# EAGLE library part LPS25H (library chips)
ST-Micro Piezoresistive pressure sensor
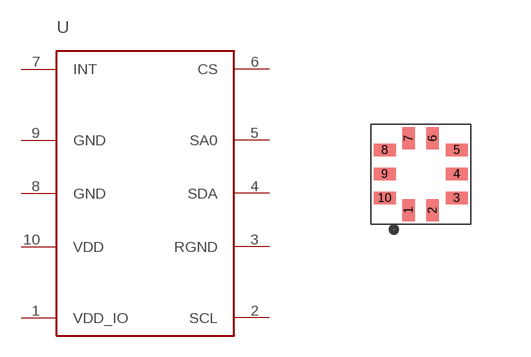
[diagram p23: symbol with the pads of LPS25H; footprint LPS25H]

Designator prefix -

## LPS25H (DIGIKEY: 497-15070-1-ND)  [LPS25H]
1  VDD_IO  pwr
2  SCL
3  RGND
4  SDA
5  SA0
6  CS
7  INT
8  GND  pwr
9  GND  pwr
10  VDD  pwr

## Footprint LPS25H (pad centres in mm)
LPS25H piezoresistive pressure sensor
smd 0.32 x 0.55: 1 -0.3,-0.9; 2 0.3,-0.9; 6 0.3,0.9; 7 -0.3,0.9
smd 0.55 x 0.32: 3 0.9,-0.6; 4 0.9,0; 5 0.9,0.6; 8 -0.9,0.6; 9 -0.9,0; 10 -0.9,-0.6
